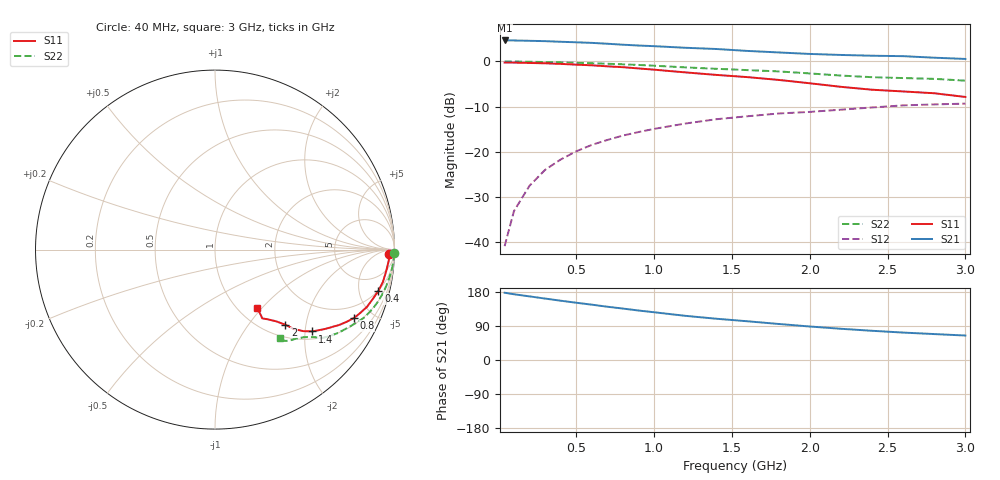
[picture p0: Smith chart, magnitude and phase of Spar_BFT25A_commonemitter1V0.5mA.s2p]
! Filename:  BFT25AC.S2P  Version:  2.0
! NXP part #: BFT25A  Date: Aug 1990
! Bias condition: Vce=1V, Ic=0.5mA
#  MHz  S  MA  R  50
! Freq  S11  S21  S12  S22  !GUM [dB]
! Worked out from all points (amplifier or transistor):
!   21 points, 40 MHz to 3 GHz, reference 50 ohm
!   highest |S21| = 4.6 dB at 40 MHz (marker M1)
!   |S21| within 3 dB of that: start of sweep to 2.014 GHz
!   unconditionally stable (mu >= 1): 2.626 GHz to end of sweep
!   at 300 MHz: K = 0.17, MSG = 14.2 dB, |S12| = -24.0 dB
!   at 1 GHz: K = 0.50, MSG = 9.2 dB, |S12| = -14.9 dB
!   at 3 GHz: K = 1.09, MAG = 3.1 dB, |S12| = -9.3 dB
!   S11 on the Smith chart (normalised r, x): 40 MHz: 38, -34; 400 MHz: 1.94, -7.54; 800 MHz: 1.30, -3.89; 1.4 GHz: 1.19, -2.19; 2 GHz: 1.23, -1.53; 3 GHz: 1.21, -0.95
40  0.971 -1.5  1.706 177.5  0.009 85.6  0.998 -1.2
100  0.97 -3.7  1.706 173.5  0.022 85.9  0.997 -3.1
200  0.961 -7.3  1.691 167.9  0.042 84.5  0.992 -6.1
300  0.953 -10.8  1.676 162.1  0.063 81.8  0.984 -9.1
400  0.939 -14.2  1.65 156.5  0.082 79.4  0.975 -12.1
500  0.921 -17.4  1.628 151.1  0.101 77.3  0.965 -14.9
600  0.905 -20.6  1.604 146.0  0.119 75.0  0.954 -17.5
700  0.882 -23.7  1.569 140.6  0.135 73.1  0.942 -19.9
800  0.863 -26.2  1.531 135.7  0.151 70.8  0.928 -22.2
900  0.836 -28.8  1.499 130.6  0.165 69.1  0.914 -24.4
1000  0.81 -31.2  1.475 126.0  0.179 67.0  0.896 -26.4
1200  0.756 -35.8  1.416 116.6  0.205 63.3  0.859 -30.4
1400  0.709 -40.0  1.372 108.9  0.229 60.6  0.828 -34.1
1600  0.67 -42.7  1.306 102.2  0.247 58.4  0.801 -37.0
1800  0.624 -45.2  1.257 95.1  0.265 56.4  0.775 -39.4
2000  0.573 -46.9  1.21 88.4  0.276 53.7  0.736 -41.5
2200  0.523 -49.7  1.179 82.4  0.292 51.4  0.697 -44.4
2400  0.486 -53.0  1.156 77.1  0.309 49.5  0.669 -48.0
2600  0.465 -55.5  1.143 72.4  0.326 48.3  0.654 -51.0
2800  0.444 -55.0  1.099 68.4  0.334 47.4  0.641 -52.5
3000  0.404 -54.2  1.065 64.6  0.341 46.8  0.612 -53.6
